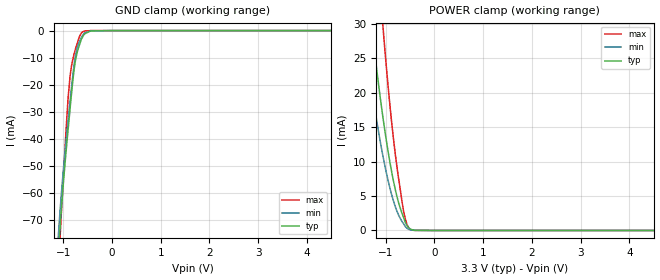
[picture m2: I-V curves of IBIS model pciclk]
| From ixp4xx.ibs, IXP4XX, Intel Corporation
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[Model]   pciclk
Model_type   Input
Vinl = 990.000mV
Vinh = 1.65V
|   typ   min   max
C_comp   3.000pF   2.700pF   3.300pF
[Voltage Range]   3.300V   3.135V   3.465V
[Temperature Range]   25.0   110.0   -40.0
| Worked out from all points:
|   GND clamp passes 1 mA (typ) near -0.54 V on its own axis
|   POWER clamp passes 1 mA (typ) near -0.59 V on its own axis
[GND Clamp]
|   Voltage   I(typ)   I(min)   I(max)
-3.3V     -1.837A    -1.782A    -2.142A
-1.11V    -85.01mA   -78.04mA   -93.41mA
-1.065V   -72.56mA   -66.27mA   -76.24mA
-1.06V    -71.11mA   -65.16mA   -74.6mA
-925mV    -41.22mA   -37.4mA    -31.6mA
-860mV    -28.8mA    -26.04mA   -16.75mA
-790mV    -16.27mA   -14.37mA   -9.57mA
-750mV    -11.01mA   -9.296mA   -6.861mA
-675mV    -5.754mA   -4.387mA   -2.478mA
-580mV    -1.626mA   -1.201mA   -252.6uA
0V        -56.89nA   -17.57nA   -32.79pA
6.595V    0A         0A         0A
[POWER Clamp]
|   Voltage   I(typ)   I(min)   I(max)
-3.3V     221.1mA    178.3mA    345.2mA
-1.5V     44.33mA    31.93mA    76.54mA
-1.44V    39.94mA    28.54mA    69.34mA
-1.27V    28.47mA    19.76mA    50.25mA
-1.06V    16.5mA     10.87mA    29.8mA
-1.045V   15.76mA    10.32mA    28.49mA
-890mV    8.924mA    5.478mA    16.42mA
-770mV    4.917mA    2.796mA    9.212mA
-635mV    1.89mA     986.7uA    2.845mA
-570mV    776uA      354.8uA    984.2uA
-515mV    310.8uA    129.8uA    274uA
6.595V    0A         0A         0A
